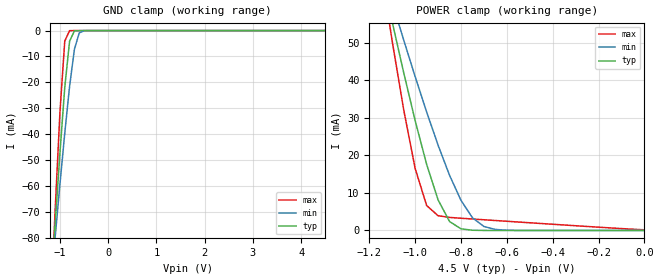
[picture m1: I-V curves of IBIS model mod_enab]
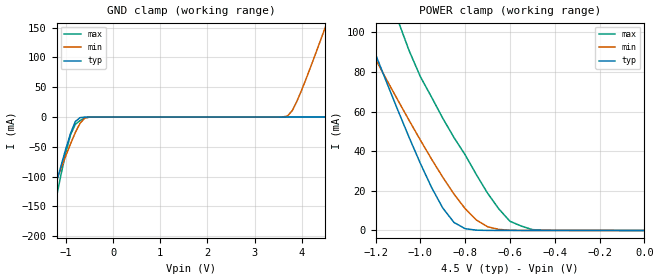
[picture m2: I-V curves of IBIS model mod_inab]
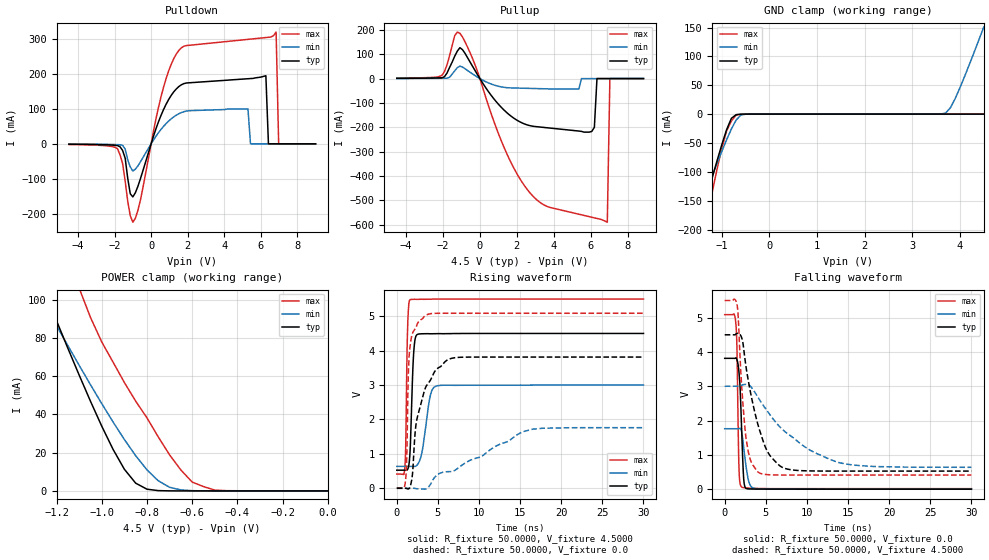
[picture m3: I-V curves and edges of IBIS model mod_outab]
| IBIS (I/O, Buffer, Information, Specification) Model, officially
| electronic behavioral standard for Buffer structures of digital pins.
[IBIS ver]  4.0
[File name] 54ac245_4v5_rev1.ibs
[File Rev]  1.0
[Date]   30 July 2013
[Source]   CAD & Design Solution (Catania) - STMicroelectronics
[Notes]
  (Note1)  54AC245 device has bidiretional behavioral that can be defined
   considering two Component structures:
   Component 54AC245AB describes the device when TR input is High
   -->  Bus A Data to Bus B
   Component 54AC245BA describes the device when TR input is Low
   -->  Bus B Data to Bus A
  (Note2)  This IBIS model is the model of the product with package
   (Flat20 package elements);
  (Note3)  This IBIS model is extracted with nominal 4.5V power supply
   (min:3.0V, typ:4.5V, max:5.5V);
  (Note4)  This model has few Warnings about the non-monotonicity
   of I-V curves, but they are not indicative of problems
   inside the model;
[Copyright] (c) 2013 STMicroelectronics
|   Component 54AC245AB
[Component] 54AC245AB
[Manufacturer] STMicroelectronics
[Package]
| variable   typ   min   max
R_pkg   0.0   0.0   0.0
L_pkg   0.0H   0.0H   0.0H
C_pkg   0.0F   0.0F   0.0F
[Pin]   signal_name   model_name   R_pin   L_pin   C_pin
TR   TR   mod_enab   178.9m   6.2nH   1.2pF
A0   A0   mod_inab   182.5m   6.3nH   1.2pF
A1   A1   mod_inab   114.4m   3.5nH   1.3pF
A2   A2   mod_inab   79.1m   2.3nH   0.9pF
A3   A3   mod_inab   75.8m   2.2nH   0.8pF
A4   A4   mod_inab   75.8m   2.2nH   0.8pF
A5   A5   mod_inab   84.5m   2.4nH   0.9pF
A6   A6   mod_inab   116.2m   3.6nH   1.3pF
A7   A7   mod_inab   178.9m   6.2nH   1.2pF
GND   GND   GND   117.4m   4.4nH   1.2pF
B7   B7   mod_outab   178.9m   6.2nH   1.2pF
B6   B6   mod_outab   189.6m   6.6nH   1.2pF
B5   B5   mod_outab   125.1m   3.9nH   1.3pF
B4   B4   mod_outab   86.3m   2.5nH   0.9pF
B3   B3   mod_outab   79.4m   2.3nH   0.8pF
B2   B2   mod_outab   75.8m   2.2nH   0.8pF
B1   B1   mod_outab   75.6m   2.1nH   0.9pF
B0   B0   mod_outab   89.3m   2.7nH   1.3pF
OE   OE   mod_enab   184.3m   6.4nH   1.2pF
VCC   VCC   POWER   118.0m   4.4nH   1.2pF
|   Component 54AC245BA
[Component]  54AC245BA
[Manufacturer] STMicroelectronics
[Package]
| variable  typ   min   max
R_pkg   0.0   0.0   0.0
L_pkg   0.0H   0.0H   0.0H
C_pkg   0.0F   0.0F   0.0F
[Pin]  signal_name   model_name   R_pin   L_pin   C_pin
TR   TR   mod_enba   178.9m   6.2nH   1.2pF
A0   A0   mod_inba   182.5m   6.3nH   1.2pF
A1   A1   mod_inba   114.4m   3.5nH   1.3pF
A2   A2   mod_inba   79.1m   2.3nH   0.9pF
A3   A3   mod_inba   75.8m   2.2nH   0.8pF
A4   A4   mod_inba   75.8m   2.2nH   0.8pF
A5   A5   mod_inba   84.5m   2.4nH   0.9pF
A6   A6   mod_inba   116.2m   3.6nH   1.3pF
A7   A7   mod_inba   178.9m   6.2nH   1.2pF
GND   GND   GND   117.4m   4.4nH   1.2pF
B7   B7   mod_outba   178.9m   6.2nH   1.2pF
B6   B6   mod_outba   189.6m   6.6nH   1.2pF
B5   B5   mod_outba   125.1m   3.9nH   1.3pF
B4   B4   mod_outba   86.3m   2.5nH   0.9pF
B3   B3   mod_outba   79.4m   2.3nH   0.8pF
B2   B2   mod_outba   75.8m   2.2nH   0.8pF
B1   B1   mod_outba   75.6m   2.1nH   0.9pF
B0   B0   mod_outba   89.3m   2.7nH   1.3pF
OE   OE   mod_enba   184.3m   6.4nH   1.2pF
VCC   VCC   POWER   118.0m   4.4nH   1.2pF
| Models and submodels in the file (6): mod_enab (Input), mod_inab (Input), mod_outab (3-state), mod_enba (Input), mod_inba (Input), mod_outba (3-state)
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|   Model mod_en
[Model]   mod_enab
Model_type Input
Vinl   =   1.3500V
Vinh   =   3.1500V
C_comp   0.532pF   NA   NA
[Temperature Range]   25.0000   0.1250k   -55.0000
[Voltage Range]   4.5000V   3.0000V   5.5000V
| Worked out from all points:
|   GND clamp passes 1 mA (typ) near -0.72 V on its own axis
|   POWER clamp passes 1 mA (typ) near -0.81 V on its own axis
[GND_clamp]
|Voltage   I(typ)   I(min)   I(max)
-4.5V     -1.124A    -840.2mA   -1.572A
-1.2V     -103.9mA   -101mA     -110.9mA
-1.1V     -75.02mA   -79.97mA   -69.86mA
-1V       -47.28mA   -59.4mA    -31.62mA
-900mV    -22mA      -39.68mA   -4.06mA
-800mV    -4.119mA   -21.58mA   -32.26uA
-700mV    -138.4uA   -7.262mA   -158.5nA
-600mV    -2.872uA   -891.6uA   -788.3pA
-500mV    -58.62nA   -53.9uA    -15.8pA
4.5V      8.75pA     6.644pA    9.881pA
[POWER_clamp]
|Voltage   I(typ)   I(min)   I(max)
-4.5V     1.102A     819.1mA    1.549A
-1.15V    69.48mA    71.05mA    69.93mA
-1.1V     55.55mA    60.82mA    50.42mA
-1.05V    42.07mA    50.78mA    32.16mA
-1V       29.27mA    41.01mA    16.51mA
-950mV    17.63mA    31.61mA    6.658mA
-900mV    8.153mA    22.74mA    3.935mA
-850mV    2.387mA    14.71mA    3.483mA
-800mV    435.6uA    8.024mA    3.262mA
-750mV    65.2uA     3.376mA    3.059mA
-700mV    9.379uA    1.056mA    2.857mA
0V        9pA        43.85pA    176uA
|   Model mod_in
[Model]   mod_inab
Model_type Input
Vinl   =   1.3500V
Vinh   =   3.1500V
C_comp   3.517pF   NA   NA
[Temperature Range]   25.0000   0.1250k   -55.0000
[Voltage Range]   4.5000V   3.0000V   5.5000V
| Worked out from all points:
|   GND clamp passes 1 mA (typ) near -0.70 V on its own axis
|   POWER clamp passes 1 mA (typ) near -0.80 V on its own axis
[GND_clamp]
|Voltage   I(typ)   I(min)   I(max)
-4.5V     -1.129A    -845.6mA   -1.584A
-1.7V     -259.6mA   -215.1mA   -344.2mA
-1.6V     -229.1mA   -193mA     -301.2mA
-1.5V     -198.8mA   -171.1mA   -258.4mA
-1.4V     -168.7mA   -149.2mA   -216.2mA
-1.3V     -138.8mA   -127.6mA   -174.5mA
-900mV    -26.79mA   -44.34mA   -28.98mA
-700mV    -976uA     -10.21mA   -5.9mA
-500mV    -12uA      -127.7uA   -211uA
3.7V      89.43pA    1.897mA    5.074pA
3.9V      94.16pA    26.87mA    5.078pA
4.5V      112.8pA    150.7mA    5.087pA
[POWER_clamp]
|Voltage   I(typ)   I(min)   I(max)
-4.5V     1.107A     824.5mA    1.575A
-1.3V     118.1mA    107.6mA    178.8mA
-1.25V    103.4mA    96.95mA    159.5mA
-1.1V     60.56mA    65.66mA    106mA
-950mV    21.72mA    36.02mA    67.3mA
-900mV    11.32mA    26.87mA    56.66mA
-850mV    4.056mA    18.4mA     46.92mA
-750mV    159.2uA    5.291mA    28.18mA
-700mV    29.54uA    1.897mA    18.82mA
-600mV    1.685uA    128.9uA    4.628mA
-500mV    160.8nA    7.103uA    429uA
0V        112.8pA    2.644nA    186.4pA
|   Model mod_outab
[Model]   mod_outab
Model_type 3-state
Enable   Active-Low
Vmeas  =   2.25V
Rref   =   500
Cref   =   50pF
C_comp   3.517pF   NA   NA
[Temperature Range]   25.0000   0.1250k   -55.0000
[Voltage Range]   4.5000V   3.0000V   5.5000V
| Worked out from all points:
|   slope of the pulldown table from 0 to 0.675 V, typ, clamps not added: 6.92 ohm
|   slope of the pullup table from 0 to 0.675 V, typ, clamps not added: 8.98 ohm
|   GND clamp passes 1 mA (typ) near -0.70 V on its own axis
|   POWER clamp passes 1 mA (typ) near -0.80 V on its own axis
|   rising waveform, R_fixture 50.0000, V_fixture 4.5000: 20-80 % time 340ps typ, 829ps min, 195ps max; typ from 0.527 V to 4.5 V
|   rising waveform, R_fixture 50.0000, V_fixture 0.0: 20-80 % time 1.82ns typ, 9.08ns min, 364ps max; typ from 0 V to 3.81 V
|   falling waveform, R_fixture 50.0000, V_fixture 0.0: 20-80 % time 360ps typ, 588ps min, 200ps max; typ from 3.81 V to 0 V
|   falling waveform, R_fixture 50.0000, V_fixture 4.5000: 20-80 % time 2.28ns typ, 6.15ns min, 882ps max; typ from 4.5 V to 0.527 V
[Pulldown]
|Voltage   I(typ)   I(min)   I(max)
-4.5V     -1.1mA     -680uA     -2mA
-1.84V    -4.97mA    -2.36mA    -13.95mA
-1V       -152mA     -78mA      -224.4mA
680mV     98.1mA     49.9mA     161.9mA
1.52V     164.1mA    86.21mA    267.6mA
5.3V      186.4mA    100mA      299.2mA
5.44V     186.9mA    0A         299.9mA
6.28V     195mA      0A         304.4mA
6.42V     0A         0A         305.1mA
6.84V     0A         0A         320mA
6.98V     0A         0A         0A
9V        0A         0A         0A
[Pullup]
|Voltage   I(typ)   I(min)   I(max)
-4.5V     1mA        440uA      1.9mA
-2.06V    3.34mA     1.31mA     12.89mA
-1.36V    92.46mA    32mA       177mA
-1.08V    127mA      51mA       186mA
1.02V     -106.7mA   -31.88mA   -229.1mA
2.56V     -190.3mA   -40.04mA   -455.1mA
6.06V     -217mA     0A         -569.7mA
6.2V      -200mA     0A         -572.2mA
6.34V     0A         0A         -574.7mA
6.9V      0A         0A         -590mA
7.04V     0A         0A         0A
8.86V     0A         0A         0A
[GND_clamp]
|Voltage   I(typ)   I(min)   I(max)
-4.5V     -1.129A    -845.6mA   -1.584A
-1.7V     -259.6mA   -215.1mA   -344.2mA
-1.6V     -229.1mA   -193mA     -301.2mA
-1.5V     -198.8mA   -171.1mA   -258.4mA
-1.4V     -168.7mA   -149.2mA   -216.2mA
-1.3V     -138.8mA   -127.6mA   -174.5mA
-900mV    -26.79mA   -44.34mA   -28.98mA
-700mV    -976uA     -10.21mA   -1.6mA
-500mV    -12uA      -127.7uA   -211uA
3.7V      89.43pA    1.897mA    5.074pA
3.9V      94.16pA    26.87mA    5.078pA
4.5V      112.8pA    150.7mA    5.087pA
[POWER_clamp]
|Voltage   I(typ)   I(min)   I(max)
-4.5V     1.107A     824.5mA    1.575A
-1.3V     118.1mA    107.6mA    178.8mA
-1.25V    103.4mA    96.95mA    159.5mA
-1.1V     60.56mA    65.66mA    106mA
-950mV    21.72mA    36.02mA    67.3mA
-900mV    11.32mA    26.87mA    56.66mA
-850mV    4.056mA    18.4mA     46.92mA
-750mV    159.2uA    5.291mA    28.18mA
-700mV    29.54uA    1.897mA    18.82mA
-600mV    1.685uA    128.9uA    4.628mA
-500mV    160.8nA    7.103uA    429uA
0V        112.8pA    2.644nA    186.4pA
[Ramp]
| variable   typ   min   max
dV/dt_r  2.2880/1.8481n   1.0572/8.9276n   3.0429/0.3932n
dV/dt_f  2.3845/2.2731n   1.4184/6.1209n   3.0523/0.9226n
R_load = 50.0000
[Rising Waveform]
R_fixture= 50.0000
V_fixture= 4.5000
V_fixture_min= 3.0000
V_fixture_max= 5.5000
|time   V(typ)   V(min)   V(max)
0s        526.6mV    636.6mV    411.9mV
990ps     526.6mV    636.6mV    623.8mV
1.08ns    527.5mV    636.6mV    1.16V
1.29ns    540mV      636.6mV    4.442V
1.59ns    965.8mV    636.6mV    5.476V
2.04ns    3.881V     637mV      5.492V
2.49ns    4.469V     681mV      5.49V
4.11ns    4.49V      2.724V     5.497V
4.83ns    4.493V     2.972V     5.499V
30ns      4.5V       3V         5.499V
[Rising Waveform]
R_fixture= 50.0000
V_fixture= 0.0
V_fixture_min= 0.0
V_fixture_max= 0.0
|time   V(typ)   V(min)   V(max)
0s        187pV      296.7pV    15.22mV
1.11ns    1.45mV     323.3nV    333.9mV
1.23ns    -8.547mV   992.3nV    1.042V
1.41ns    -20.13mV   2.744uV    3.36V
1.74ns    152.4mV    -67.27uV   4.338V
2.34ns    1.858V     -9.879mV   4.676V
3.48ns    2.917V     -24.73mV   5.02V
6.36ns    3.754V     484.8mV    5.087V
15.33ns   3.814V     1.644V     5.087V
30ns      3.814V     1.762V     5.087V
[Falling Waveform]
R_fixture= 50.0000
V_fixture= 0.0
V_fixture_min= 0.0
V_fixture_max= 0.0
|time   V(typ)   V(min)   V(max)
0s        3.814V     1.762V     5.087V
1.35ns    3.828V     1.762V     4.85V
1.5ns     3.77V      1.761V     4.002V
1.68ns    3.538V     1.761V     1.185V
1.77ns    3.321V     1.767V     404mV
2.07ns    1.667V     1.661V     60.01mV
2.31ns    296.5mV    1.218V     42.95mV
2.73ns    12.48mV    457.6mV    37.26mV
4.05ns    2.768mV    11.42mV    19.96mV
30ns      -45.59nV   4.836uV    15.22mV
[Falling Waveform]
R_fixture= 50.0000
V_fixture= 4.5000
V_fixture_min= 3.0000
V_fixture_max= 5.5000
|time   V(typ)   V(min)   V(max)
0s        4.5V       3V         5.499V
1.47ns    4.539V     3V         5.41V
1.62ns    4.545V     2.999V     5.125V
2.13ns    4.363V     3.037V     2.777V
2.61ns    3.538V     3.052V     1.462V
3.21ns    2.734V     2.979V     799.5mV
4.11ns    1.825V     2.654V     489.4mV
6.93ns    645.4mV    1.763V     412.7mV
13.41ns   527.1mV    811mV      411.9mV
30ns      526.6mV    636.9mV    411.9mV
